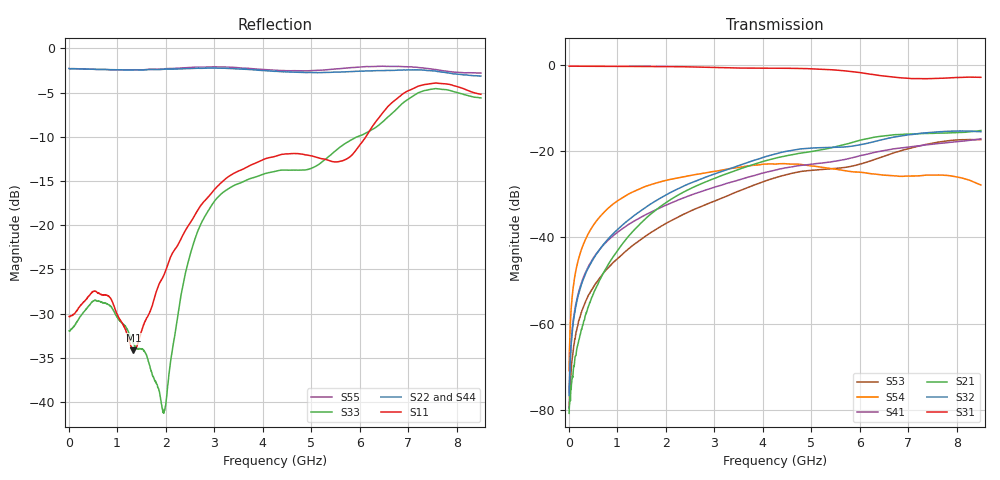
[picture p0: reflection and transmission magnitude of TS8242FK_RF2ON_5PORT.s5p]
! Created with skrf (http://scikit-rf.org).
# Hz S RI R 50.0
!freq ReS11 ImS11 ReS12 ImS12 ReS13 ImS13
! ReS14 ImS14 ReS15 ImS15
! ReS21 ImS21 ReS22 ImS22 ReS23 ImS23
! ReS24 ImS24 ReS25 ImS25
! ReS31 ImS31 ReS32 ImS32 ReS33 ImS33
! ReS34 ImS34 ReS35 ImS35
! ReS41 ImS41 ReS42 ImS42 ReS43 ImS43
! ReS44 ImS44 ReS45 ImS45
! ReS51 ImS51 ReS52 ImS52 ReS53 ImS53
! ReS54 ImS54 ReS55 ImS55
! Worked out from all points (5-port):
!   1601 points, 10 MHz to 8.5 GHz, reference 50 ohm
!   strongest paths, dB at 10 MHz, 2.132 GHz, 4.255 GHz, 6.378 GHz, 8.5 GHz:
!     S31: -0.3, -0.4, -0.7, -2.4, -2.8
!     S32: -76.7, -29.4, -20.7, -17.5, -15.5
!     S21: -80.8, -31.0, -21.6, -16.6, -15.2
!     S41: -76.0, -31.9, -24.4, -20.1, -17.1
!     S54: -70.9, -26.5, -23.0, -25.4, -27.8
!     S53: -79.7, -36.0, -26.2, -21.6, -17.3
!   lowest |S11| = -34.2 dB at 1.337 GHz (marker M1), VSWR 1.04, Z = 50.5 - j1.89 ohm
!   |S11| at or under -10 dB: start of sweep to 6.128 GHz
